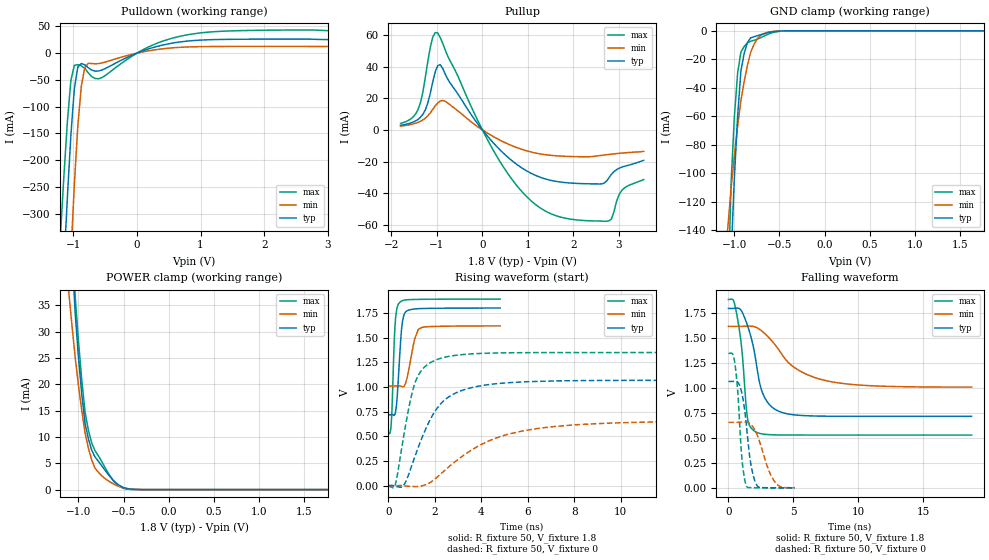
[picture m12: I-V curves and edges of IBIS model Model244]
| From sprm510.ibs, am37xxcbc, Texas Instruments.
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| Model based on original model for BQ18OMAPSMART1HYFBPB_SSBHV
|   Sub model PB_VS10L00_PUPD0_1P8
[model]   Model244
|[Input Load]   PI
|[Output Drive] SC10LB00
|Voltage   1.8V
|Mode   I/O
Model_type   I/O
Polarity   Non-Inverting
Enable   Active-Low
Vinl =  0.63
Vinh =  1.17
Cref =  15pF
Rref =  100.0000M
Vref =  0V
Vmeas =  0.9
C_comp   1.429432p   1.270657p   1.602015p
[Model Spec]
Vinl   0.63   0.567   0.6615
Vinh   1.17   1.053   1.2285
[Temperature Range]   25   125   -40
[Voltage Range]   1.8   1.62   1.89
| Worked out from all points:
|   slope of the pulldown table from 0 to 0.27 V, typ, clamps not added: 24.3 ohm
|   slope of the pullup table from 0 to 0.27 V, typ, clamps not added: 29.7 ohm
|   GND clamp passes 1 mA (typ) near -0.60 V on its own axis
|   POWER clamp passes 1 mA (typ) near -0.56 V on its own axis
|   rising waveform, R_fixture 50, V_fixture 1.8: 20-80 % time 179ps typ, 308ps min, 126ps max; typ from 0.718 V to 1.8 V
|   rising waveform, R_fixture 50, V_fixture 0: 20-80 % time 1.34ns typ, 2.9ns min, 711ps max; typ from 0 V to 1.07 V
|   falling waveform, R_fixture 50, V_fixture 1.8: 20-80 % time 1.11ns typ, 2.94ns min, 574ps max; typ from 1.8 V to 0.718 V
|   falling waveform, R_fixture 50, V_fixture 0: 20-80 % time 591ps typ, 1.02ns min, 414ps max; typ from 1.07 V to 0 V
[POWER_clamp]
-1.8V     362.5mA    191.4mA    412.8mA
-1.109V   56.69mA    37.71mA    60.38mA
-1.073V   44.6mA     31.22mA    47.8mA
-1.036V   33.44mA    25.04mA    36.59mA
-1V       24.98mA    19.72mA    28.06mA
-963.6mV  18.03mA    14.96mA    20.78mA
-927.3mV  12.59mA    10.77mA    14.74mA
-890.9mV  9.653mA    7.899mA    11.31mA
-818.2mV  6.214mA    4.114mA    7.414mA
-636.4mV  2.183mA    1.307mA    2.238mA
-418.2mV  83.85uA    105.2uA    35.14uA
1.764V    -1.228nA   -79.12nA   -1.453nA
[Pulldown]
-1.8V     -1.718A    -2.61A     -1.406A
-1.2V     -527.4mA   -844.5mA   -339.9mA
-1.145V   -396mA     -683.1mA   -229.1mA
-1.091V   -269mA     -526.7mA   -127.5mA
-1.036V   -153.6mA   -378.9mA   -51.17mA
-981.8mV  -66.34mA   -245.6mA   -22.67mA
-927.3mV  -26mA      -136.2mA   -21.54mA
-872.7mV  -19.34mA   -61.98mA   -23.69mA
-763.6mV  -27.2mA    -19.05mA   -36.72mA
-545.5mV  -31.39mA   -18.17mA   -45.46mA
872.7mV   23.46mA    11.88mA    35.92mA
3.545V    25.34mA    12.51mA    41.58mA
[Pullup]
-1.8V     2.903mA    2.423mA    4.112mA
-1.418V   6.595mA    4.711mA    12.64mA
-1.255V   12.69mA    7.42mA     33.23mA
-1.091V   30.4mA     13mA       58.69mA
-981.8mV  40.63mA    17.02mA    61.3mA
-818.2mV  35.38mA    18.12mA    50.59mA
272.7mV   -9.18mA    -4.728mA   -14.55mA
1.255V    -29.75mA   -15.09mA   -48.97mA
2.564V    -34.17mA   -16.31mA   -57.57mA
2.782V    -30.25mA   -15.5mA    -57.48mA
3.055V    -23.63mA   -14.68mA   -38.61mA
3.545V    -19.25mA   -13.56mA   -31.41mA
[GND_clamp]
-1.8V     -2.82A     -1.192A    -3.165A
-1.073V   -235.7mA   -138.4mA   -192.1mA
-1.036V   -159.5mA   -110.8mA   -107.5mA
-1V       -103.8mA   -87.85mA   -60.67mA
-963.6mV  -60mA      -67.28mA   -29.8mA
-927.3mV  -28.21mA   -49.08mA   -14.9mA
-890.9mV  -15.9mA    -35.48mA   -10.99mA
-854.5mV  -8.138mA   -24.07mA   -8.449mA
-818.2mV  -4.924mA   -14.85mA   -7.266mA
-709.1mV  -2.784mA   -3.064mA   -4.883mA
-563.6mV  -570.2uA   -404.5uA   -1.092mA
1.764V    -11.02pA   583.5nA    3.035nA
[Ramp]
dV/dt_f  0.6514733/1.10759n   0.3680067/2.970961n   0.8183131/0.5759545n
dV/dt_r  0.6510765/1.339497n   0.4007893/2.925416n   0.823178/0.7143078n
R_load = 50
[Rising Waveform]
R_fixture = 50
V_fixture = 1.8
V_fixture_min = 1.62
V_fixture_max = 1.89
0s        717.6mV    1.009V     531.7mV
126ps     718.3mV    1.009V     635.8mV
252ps     712.4mV    1.009V     1.458V
306ps     744.3mV    1.009V     1.683V
459ps     1.2V       1.011V     1.848V
612ps     1.669V     1V         1.875V
792ps     1.77V      1.079V     1.883V
1.134ns   1.79V      1.486V     1.887V
1.44ns    1.795V     1.603V     1.888V
4.815ns   1.8V       1.618V     1.89V
[Rising Waveform]
R_fixture = 50
V_fixture = 0
V_fixture_min = 0
V_fixture_max = 0
0s        -257.2uV   61.34uV    -2.41mV
297ps     -8.432mV   -421.6uV   9.092mV
693ps     14.14mV    -3.21mV    546.4mV
999ps     196.8mV    -8.477mV   916.9mV
1.197ns   329.4mV    -10.47mV   1.072V
1.764ns   651.5mV    26.66mV    1.239V
2.286ns   837.2mV    123.9mV    1.292V
4.212ns   1.02V      440.6mV    1.341V
6.462ns   1.057V     580.1mV    1.348V
20.11ns   1.067V     655.8mV    1.349V
[Falling Waveform]
R_fixture = 50
V_fixture = 1.8
V_fixture_min = 1.62
V_fixture_max = 1.89
0s        1.8V       1.62V      1.89V
405ps     1.801V     1.62V      1.875V
801ps     1.801V     1.62V      1.619V
1.026ns   1.769V     1.62V      1.394V
1.494ns   1.618V     1.622V     676.8mV
2.088ns   1.293V     1.613V     562.8mV
2.844ns   892.3mV    1.542V     537mV
4.221ns   752.6mV    1.319V     530.3mV
8.217ns   718.3mV    1.058V     529.8mV
18.71ns   717.6mV    1.011V     529.8mV
[Falling Waveform]
R_fixture = 50
V_fixture = 0
V_fixture_min = 0
V_fixture_max = 0
0s        1.068V     657.3mV    1.349V
351ps     1.068V     657.7mV    1.336V
522ps     1.071V     657.5mV    1.222V
738ps     1.056V     657.5mV    924.3mV
1.044ns   944mV      660mV      285.2mV
1.395ns   610mV      659.3mV    14.52mV
1.746ns   222.1mV    633mV      1.671mV
2.196ns   23.91mV    535.8mV    277.7uV
3.546ns   360.6uV    64.32mV    8.366uV
5.112ns   66.03uV    1.63mV     937.1nV
